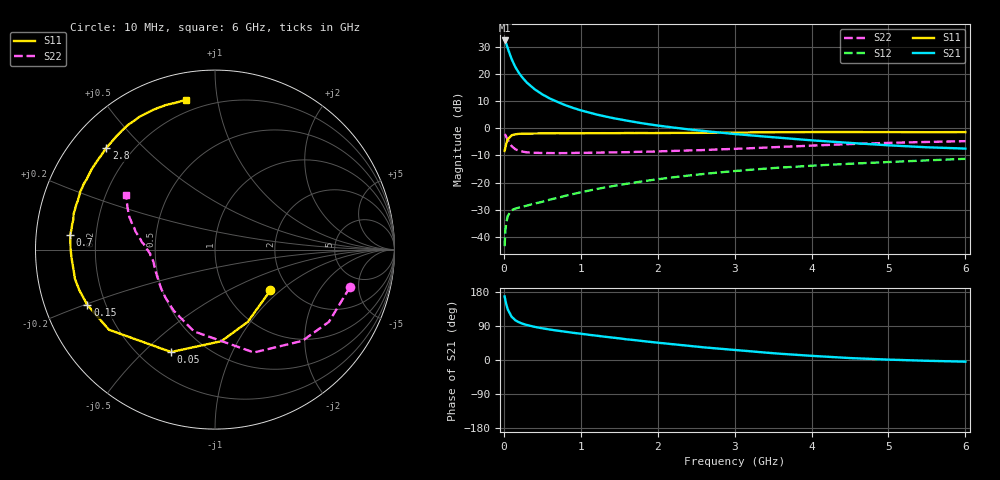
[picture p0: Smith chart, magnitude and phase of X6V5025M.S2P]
! SIEMENS Small Signal Semiconductors
! BFP193W
! Si NPN RF Bipolar Junction Transistor in SOT343
! VCE = 0.5 V  IC = 25 mA
! Common Emitter S-Parameters:  April 1994
# GHz  S  MA  R  50
!  f  S11  S21  S12  S22
! GHz  MAG  ANG  MAG  ANG  MAG  ANG  MAG  ANG
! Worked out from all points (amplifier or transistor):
!   40 points, 10 MHz to 6 GHz, reference 50 ohm
!   highest |S21| = 32.3 dB at 10 MHz (marker M1)
!   |S21| within 3 dB of that: start of sweep to 52.03 MHz
!   unconditionally stable (mu >= 1): 506.9 MHz to end of sweep
!   at 200 MHz: K = 0.52, MSG = 24.7 dB, |S12| = -29.1 dB
!   at 1.5 GHz: K = 1.35, MAG = 8.5 dB, |S12| = -20.9 dB
!   at 6 GHz: K = 1.17, MAG = -0.6 dB, |S12| = -11.2 dB
!   S11 on the Smith chart (normalised r, x): 10 MHz: 1.61, -0.86; 50 MHz: 0.33, -0.61; 150 MHz: 0.13, -0.20; 700 MHz: 0.10, +0.05; 2.8 GHz: 0.11, +0.39; 6 GHz: 0.14, +0.82
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0.01  0.3832 -36.3  41.11 167.7  0.0068 77.1  0.7804 -15.6
0.02  0.4422 -65.6  38.89 157.7  0.0132 68.5  0.7516 -32.4
0.03  0.5115 -86.0  36.17 148.4  0.0177 61.1  0.7036 -46.3
0.05  0.6209 -113.2  29.64 133.8  0.0243 48.8  0.6126 -69.3
0.1  0.7405 -142.9  18.86 114.5  0.0311 35.1  0.4705 -104.4
0.15  0.775 -156.5  13.3 104.8  0.0334 30.8  0.4109 -124.1
0.2  0.789 -163.3  10.18 99.2  0.0349 30.5  0.3842 -136.1
0.25  0.7973 -168.2  8.269 95.3  0.0363 31.4  0.3707 -143.9
0.3  0.7961 -171.5  6.894 92.3  0.0379 33.2  0.3612 -149.7
0.4  0.8005 -176.6  5.213 87.5  0.0413 36.5  0.3537 -156.8
0.5  0.8048 179.8  4.199 83.7  0.0445 39.9  0.3515 -161.4
0.6  0.8068 176.9  3.509 80.3  0.0488 42.8  0.3501 -164.8
0.7  0.8109 174.2  3.039 77.4  0.0526 45.2  0.3494 -167.1
0.9  0.8082 169.9  2.368 71.8  0.0618 48.7  0.3517 -170.3
1.1  0.8125 165.9  1.96 66.7  0.0712 51.0  0.3546 -172.7
1.6  0.8172 156.7  1.381 54.5  0.0956 52.8  0.3632 -176.7
2.2  0.8206 146.6  1.033 41.6  0.1254 51.0  0.3831 178.7
2.8  0.8295 136.9  0.835 29.9  0.1541 47.4  0.4088 174.3
3.2  0.8372 130.8  0.742 23.1  0.1722 44.5  0.4291 170.8
4.5  0.8517 113.7  0.538 5.1  0.2227 34.4  0.5127 158.9
5.5  0.8471 105.1  0.447 -2.1  0.2567 27.7  0.5599 151.4
6  0.8503 101.0  0.423 -4.4  0.2743 24.6  0.5794 148.4
